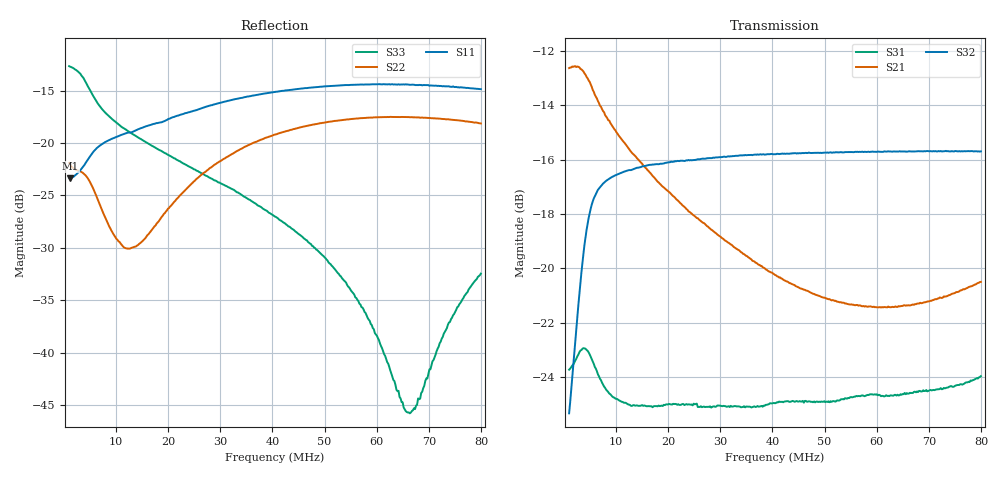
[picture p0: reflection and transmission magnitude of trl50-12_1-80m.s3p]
!transmissionline Übertrager mit 2 Würth Rohrkernen gross und 2 x 1 5 Wdgn 25 Ohm Koax  DC-Einspeisung über Mitte der Schirme
!Fri 11/May/2018 15:27:40
# HZ S MA R 50
!freq[Hz] magS11 angS11 magS12 angS12 magS13 angS13
! magS21 angS21 magS22 angS22 magS23 angS23
! magS31 angS31 magS32 angS32 magS33 angS33
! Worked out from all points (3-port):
!   401 points, 1 MHz to 80 MHz, reference 50 ohm
!   strongest paths, dB at 1 MHz, 20.75 MHz, 40.5 MHz, 60.25 MHz, 80 MHz:
!     S32: -25.3, -16.1, -15.8, -15.7, -15.7
!     S21: -12.6, -17.3, -20.2, -21.4, -20.5
!     S31: -23.7, -25.0, -25.0, -24.7, -24.0
!   lowest |S11| = -23.4 dB at 1.198 MHz (marker M1), VSWR 1.15, Z = 56.2 + j3.63 ohm
!   |S11| at or under -10 dB: start of sweep to end of sweep
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1000000  0.06829 33.1  0.2361 3.0  0.06719 -14.9
         0.2336 3.4  0.08036 158.5  0.05457 24.2
         0.06506 -15.1  0.05408 24.5  0.2327 174.7
1197500  0.06785 28.3  0.2365 0.4  0.06747 -19.8
         0.2342 0.8  0.07878 157.5  0.05736 26.0
         0.06536 -20.2  0.05663 26.4  0.2314 172.7
5147500  0.08729 -0.1  0.22 -28.1  0.06913 -100.4
         0.2179 -28.0  0.06411 110.5  0.1304 19.7
         0.06871 -101.9  0.1288 19.8  0.1764 144.0
9492500  0.1055 -27.2  0.1837 -44.6  0.05778 -145.2
         0.1814 -44.8  0.03677 54.3  0.1495 -2.8
         0.05787 -146.5  0.1477 -2.9  0.1285 137.2
1.26525e7  0.1122 -43.3  0.1667 -54.2  0.05588 -164.3
           0.1649 -54.4  0.03132 12.4  0.1532 -13.4
           0.05604 -165.4  0.1517 -13.5  0.1127 133.8
2.6675e7  0.1474 -93.4  0.123 -88.7  0.05661 140.4
          0.1213 -89.2  0.07157 -89.0  0.1614 -49.1
          0.05558 139.9  0.1592 -49.7  0.07122 119.9
4.05e7  0.1752 -132.7  0.09848 -116.8  0.05725 98.1
        0.09722 -117.5  0.1098 -132.3  0.1644 -81.5
        0.05643 97.4  0.1622 -82.2  0.04454 108.5
5.53125e7  0.1894 -167.5  0.08685 -141.2  0.05839 58.3
           0.08572 -142.1  0.1303 -167.3  0.1657 -114.9
           0.05787 57.5  0.1637 -115.8  0.01946 102.0
6.6175e7  0.1901 168.6  0.08644 -158.2  0.0589 32.4
          0.0855 -159.1  0.1331 169.8  0.166 -139.1
          0.05879 30.6  0.1642 -140.2  0.005178 160.7
8e7  0.1808 137.7  0.09548 178.3  0.06999 -6.5
     0.0944 177.1  0.124 142.2  0.166 -170.0
     0.06331 -3.0  0.1641 -171.2  0.02381 -135.6
